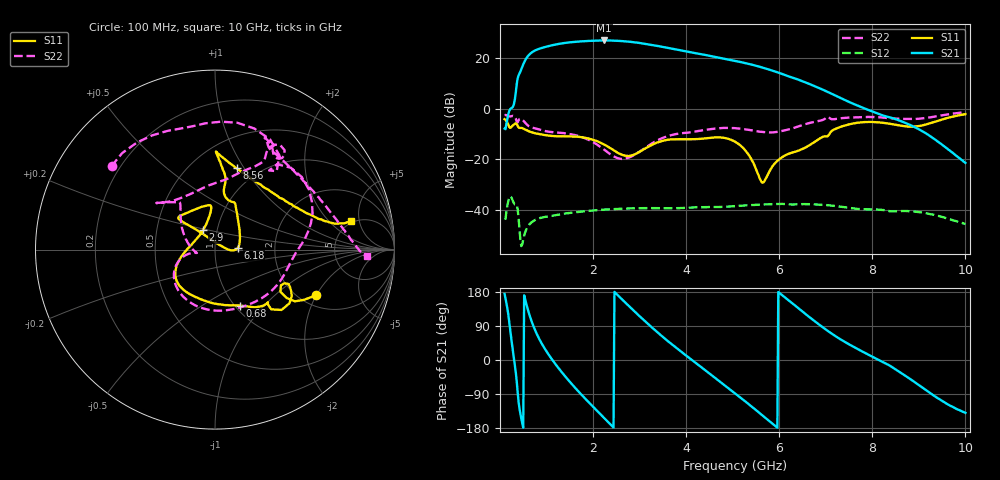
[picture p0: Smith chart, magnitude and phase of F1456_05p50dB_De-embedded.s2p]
! Integrated Device Technology
! Corporate Headquarters
! 6024 Silver Creek Valley Road
! San Jose, CA 95138  USA
! Phone:  1-408-284-8200
! Toll Free:  1-800-223-1366
! Webpage:  http://www.idt.com/
! Timing and RF Division
! 515 Groton Road, Suite 102
! Westford, MA 01886-6024
! Device:  F1456
! Description: 6-bit 0.5 dB Transmit Variable Gain Amplifier
! Frequency:  2100.0 -  2950.00 MHz
! Package:  6x6 mm Thin QFN Plastic Package: 28 pin
! State:  11
! Atten State:  5.5 dB
! Voltage:  +5.00 Volts
! Current:  216.148 mA
! Data:  The device was measured on a the F1455 evaluation board which has
!  individual transmission lines to the RF pins.  Data was collected
!  using a calibrated network analyzer.  The evaluation board was
!  de-embedded using a TRL calibration technique.
!  The reference plane is the edge of the package pin.
!  Pin  1 = CSb
!  Pin  2 = DATA
!  Pin  3 = CLK
!  Pin  4 = RSET
!  Pin  5 = GND
!  Pin  6 = RFIN  = Port 1
!  Pin  7 = GND
!  Pin  8 = NC
!  Pin  9 = NC
!  Pin 10 = NC
!  Pin 11 = NC
!  Pin 12 = NC
!  Pin 13 = NC
!  Pin 14 = /STBY
!  Pin 15 = GND
!  Pin 16 = RFOUT  = Port 2
!  Pin 17 = GND
!  Pin 18 = NC
!  Pin 19 = NC
!  Pin 20 = NC
!  Pin 21 = GND
!  Pin 22 = NC
!  Pin 23 = GND
!  Pin 24 = NC
!  Pin 25 = NC
!  Pin 26 = NC
!  Pin 27 = GND
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# GHz S dB R 50
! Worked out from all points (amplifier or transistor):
!   496 points, 100 MHz to 10 GHz, reference 50 ohm
!   highest |S21| = 26.7 dB at 2.24 GHz (marker M1)
!   |S21| within 3 dB of that: 888.8 MHz to 3.625 GHz (2.736 GHz wide, 121 % of centre)
!   unconditionally stable (mu >= 1): start of sweep to end of sweep
!   at 1.74 GHz: K = 2.32, MAG = 27.0 dB, |S12| = -40.5 dB
!   at 5.06 GHz: K = 3.92, MAG = 19.6 dB, |S12| = -38.3 dB
!   at 10 GHz: K = 123.95, MAG = -11.9 dB, |S12| = -45.3 dB
!   S11 on the Smith chart (normalised r, x): 100 MHz: 2.43, -1.99; 680 MHz: 1.05, -0.74; 2.9 GHz: 0.85, +0.19; 6.18 GHz: 1.29, +0.02; 8.56 GHz: 0.80, +0.93; 10 GHz: 4.75, +3.79
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0.1  -4.18 -24.1  -7.88 174.6  -43.14 43.7  -2.61 141.1
0.34  -5.83 -35.8  6.26 -32.2  -37.60 -145.7  -3.94 55.6
0.42  -7.61 -44.8  13.70 -128.5  -47.51 138.6  -4.13 47.2
0.54  -8.17 -55.5  18.85 160.6  -48.66 -169.3  -5.56 10.8
0.68  -9.33 -65.9  21.96 102.1  -44.66 151.3  -7.43 -10.4
0.86  -10.10 -80.7  23.54 51.7  -42.98 110.2  -8.29 -39.4
1.16  -10.83 -106.5  24.99 -5.6  -41.99 69.4  -9.32 -84.0
1.48  -10.91 -127.7  25.93 -54.6  -41.00 41.2  -9.96 -122.6
1.76  -11.27 -142.5  26.37 -92.7  -40.42 21.4  -11.22 -146.4
2.24  -14.16 -167.0  26.71 -153.2  -39.67 -7.4  -16.15 -170.3
2.54  -17.48 168.4  26.56 170.0  -39.37 -24.0  -19.56 -169.8
2.9  -17.94 122.2  25.96 127.1  -39.16 -42.9  -18.08 179.4
3.4  -13.25 96.0  24.51 71.4  -39.10 -67.4  -12.37 141.3
4.08  -12.07 110.8  22.10 4.2  -38.89 -96.2  -9.37 129.0
4.58  -11.36 135.8  20.42 -43.1  -38.71 -117.8  -7.96 139.2
5.06  -13.12 138.6  18.67 -88.7  -38.30 -138.2  -7.73 140.8
5.6  -28.04 82.5  16.28 -142.3  -37.70 -165.8  -9.13 126.2
6.18  -17.93 3.9  12.77 159.5  -37.61 159.2  -8.30 84.6
6.7  -13.84 50.4  9.24 108.2  -37.58 128.5  -5.48 63.0
8.36  -5.94 83.4  -3.38 -13.8  -40.27 53.1  -3.82 62.4
8.56  -6.58 75.2  -4.58 -29.5  -40.34 48.2  -4.00 57.4
10  -2.22 11.9  -21.33 -139.3  -45.34 -29.8  -1.46 -2.5
